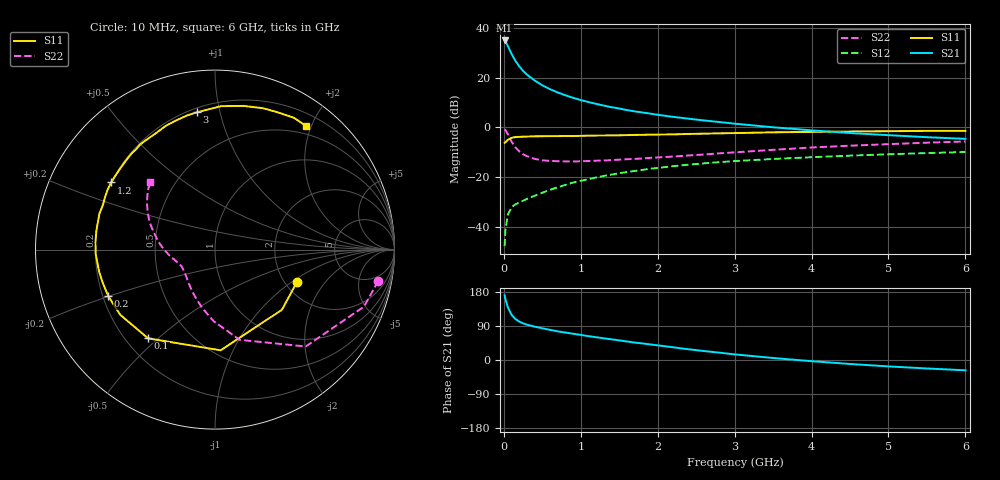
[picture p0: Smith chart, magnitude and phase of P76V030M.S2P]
! SIEMENS Small Signal Semiconductors
! BFP196
! Si NPN RF Bipolar Junction Transistor in SOT143
! VCE = 6 V  IC = 30 mA
! Common Emitter S-Parameters:  May  1996
# GHz  S  MA  R  50
!  f  S11  S21  S12  S22
! GHz  MAG  ANG  MAG  ANG  MAG  ANG  MAG  ANG
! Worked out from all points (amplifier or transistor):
!   36 points, 10 MHz to 6 GHz, reference 50 ohm
!   highest |S21| = 35.0 dB at 10 MHz (marker M1)
!   |S21| within 3 dB of that: start of sweep to 63.9 MHz
!   unconditionally stable (mu >= 1): 588.3 MHz to 4.104 GHz
!   at 250 MHz: K = 0.70, MSG = 26.1 dB, |S12| = -29.5 dB
!   at 1.4 GHz: K = 1.10, MAG = 11.7 dB, |S12| = -18.9 dB
!   at 6 GHz: K = 0.97, MSG = 2.6 dB, |S12| = -9.9 dB
!   lowest NFmin = 1.40 dB at 500 MHz
!   S11 on the Smith chart (normalised r, x): 10 MHz: 2.31, -1.10; 100 MHz: 0.29, -0.46; 200 MHz: 0.22, -0.20; 1.2 GHz: 0.20, +0.28; 3 GHz: 0.23, +0.85; 6 GHz: 0.38, +1.92
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0.01  0.491 -21.7  56.36 171.0  0.0041 83.0  0.9257 -10.9
0.02  0.5014 -42.0  53.81 161.2  0.0084 74.8  0.8893 -20.9
0.05  0.562 -86.8  44.4 140.1  0.0174 59.4  0.7394 -46.9
0.1  0.6192 -127.0  30.22 119.3  0.0248 46.2  0.5212 -74.7
0.15  0.641 -145.5  21.93 108.2  0.0285 44.0  0.3988 -91.1
0.2  0.6488 -156.4  17.06 101.4  0.0309 44.3  0.3314 -102.7
0.25  0.6526 -163.9  13.77 96.7  0.0336 45.9  0.2884 -111.9
0.3  0.6573 -169.5  11.6 93.3  0.0366 48.0  0.265 -118.7
0.4  0.6652 -177.9  8.82 88.0  0.0424 51.2  0.2343 -129.6
0.5  0.6672 176.5  7.058 83.7  0.0487 53.8  0.2194 -137.0
0.6  0.6692 171.2  5.895 79.5  0.0557 55.0  0.2126 -142.2
0.7  0.6706 166.2  5.077 75.6  0.0628 56.6  0.2098 -146.4
0.9  0.6714 158.5  3.955 69.3  0.0781 56.7  0.2078 -152.6
1.1  0.6854 150.8  3.252 63.0  0.0915 56.2  0.2121 -156.6
1.2  0.6891 147.1  2.985 60.1  0.0989 55.6  0.2149 -158.6
1.7  0.7088 131.1  2.112 46.0  0.1336 50.6  0.2336 -166.6
2.2  0.7264 117.3  1.636 33.5  0.1666 44.3  0.2602 -173.9
3  0.7715 97.4  1.195 14.8  0.2111 33.6  0.3161 172.5
3.5  0.7999 87.6  1.01 5.3  0.2329 27.1  0.3554 164.2
4.5  0.8319 71.3  0.774 -10.5  0.2715 15.6  0.4304 150.7
5.5  0.8559 59.1  0.638 -22.4  0.3057 5.0  0.495 139.2
6  0.8551 53.6  0.591 -27.2  0.3217 -0.7  0.5237 133.7
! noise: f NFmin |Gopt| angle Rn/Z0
0.5  1.4  0.4  -173  0.08
0.9  1.6  0.5  -166  0.08
1.5  2.4  0.61  -150  0.14
2  2.9  0.71  -129  0.2
